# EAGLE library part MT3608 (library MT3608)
High Efficiency 1.2MHz 2A Step Up Converter Source: Datasheet
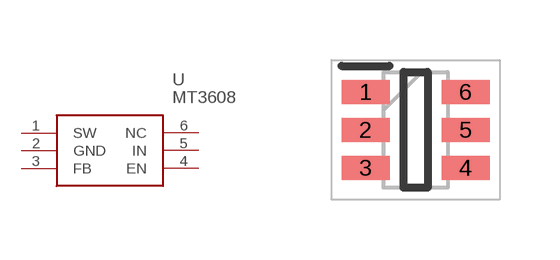
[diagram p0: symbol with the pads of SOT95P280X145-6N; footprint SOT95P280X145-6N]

Designator prefix U

## MT3608 (Description: High Efficiency 1.2MHz 2A Step Up Converter; Height: 1.45mm; Manufacturer_Name: Aerosemi; Manufacturer_Part_Number: MT3608)  [SOT95P280X145-6N]
1  SW
2  GND
3  FB
4  EN
5  IN
6  NC  nc

## Footprint SOT95P280X145-6N (pad centres in mm)
TSOT23-6/SOT23-6
smd 1.2 x 0.6: 1 -1.25,0.95; 2 -1.25,0; 3 -1.25,-0.95; 4 1.25,-0.95; 5 1.25,0; 6 1.25,0.95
